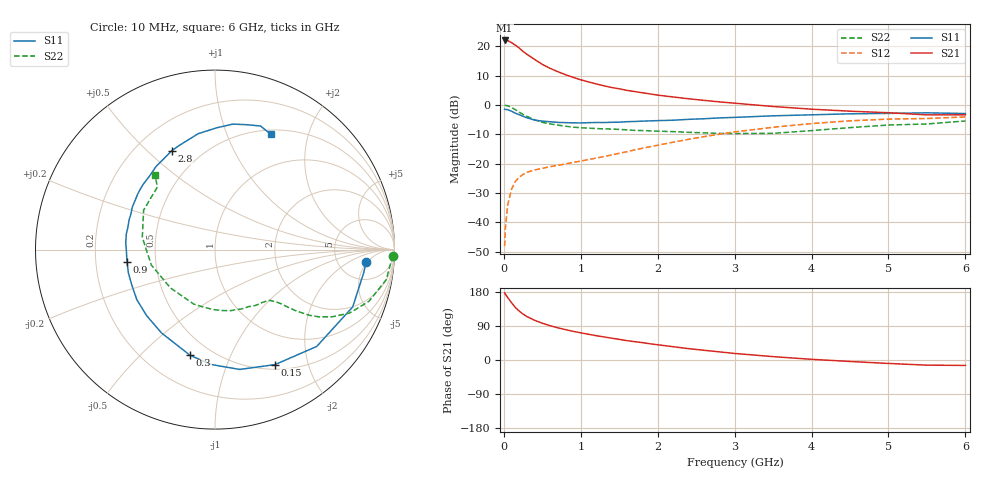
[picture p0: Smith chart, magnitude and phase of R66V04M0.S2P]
! SIEMENS Small Signal Semiconductors
! BFR193
! Si NPN RF Bipolar Junction Transistor in SOT23
! VCE = 6 V  IC = 4 mA
! Common Emitter S-Parameters:  May  1996
# GHz  S  MA  R  50
!  f  S11  S21  S12  S22
! GHz  MAG  ANG  MAG  ANG  MAG  ANG  MAG  ANG
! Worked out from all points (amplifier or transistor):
!   36 points, 10 MHz to 6 GHz, reference 50 ohm
!   highest |S21| = 22.0 dB at 10 MHz (marker M1)
!   |S21| within 3 dB of that: start of sweep to 217.5 MHz
!   unconditionally stable (mu >= 1): 968.2 MHz to 2.032 GHz
!   at 250 MHz: K = 0.36, MSG = 21.0 dB, |S12| = -23.7 dB
!   at 1.4 GHz: K = 1.08, MAG = 9.8 dB, |S12| = -17.1 dB
!   at 6 GHz: K = 0.97, MSG = 0.4 dB, |S12| = -4.1 dB
!   S11 on the Smith chart (normalised r, x): 10 MHz: 10, -5; 150 MHz: 0.56, -1.50; 300 MHz: 0.39, -0.72; 900 MHz: 0.34, -0.06; 2.8 GHz: 0.35, +0.60; 6 GHz: 0.55, +1.45
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0.01  0.846 -4.6  12.6 177.2  0.0039 84.6  0.9926 -2.0
0.02  0.838 -9.1  12.57 173.7  0.0079 85.9  0.9832 -4.0
0.05  0.831 -22.6  12.54 164.8  0.0198 78.7  0.9685 -10.0
0.1  0.7825 -43.6  11.57 151.2  0.0365 68.2  0.9046 -18.6
0.15  0.7227 -62.5  10.46 138.5  0.0496 60.3  0.8295 -25.2
0.2  0.6816 -78.4  9.343 129.0  0.0586 54.7  0.7533 -29.8
0.25  0.6405 -91.9  8.18 121.1  0.0652 50.5  0.6896 -32.9
0.3  0.605 -103.3  7.313 114.6  0.0709 47.8  0.6392 -34.9
0.4  0.5517 -122.7  5.975 104.8  0.0779 45.2  0.558 -37.3
0.5  0.5296 -136.0  4.925 97.0  0.0828 44.5  0.5046 -38.6
0.6  0.5173 -147.3  4.22 90.7  0.0886 44.5  0.4753 -39.4
0.7  0.5041 -156.7  3.703 85.0  0.0931 46.0  0.4532 -40.3
0.9  0.4953 -172.0  2.96 75.7  0.1048 49.5  0.418 -42.6
1.1  0.4986 175.7  2.472 67.9  0.117 52.8  0.402 -46.1
1.3  0.501 165.4  2.123 60.9  0.1318 55.6  0.3909 -49.9
1.6  0.5184 152.5  1.773 51.1  0.1595 58.5  0.3762 -57.1
2.2  0.5489 131.5  1.368 35.1  0.2315 58.9  0.3509 -75.8
2.8  0.6011 113.7  1.129 21.5  0.3164 53.6  0.3269 -101.4
3.5  0.6527 98.2  0.941 8.9  0.4163 42.9  0.3276 -139.4
4.5  0.7063 81.9  0.783 -3.9  0.5363 25.3  0.4107 170.4
5.5  0.7338 69.8  0.677 -13.6  0.5871 7.5  0.4741 132.6
6  0.714 64.2  0.68 -14.3  0.6252 2.4  0.5333 128.8
